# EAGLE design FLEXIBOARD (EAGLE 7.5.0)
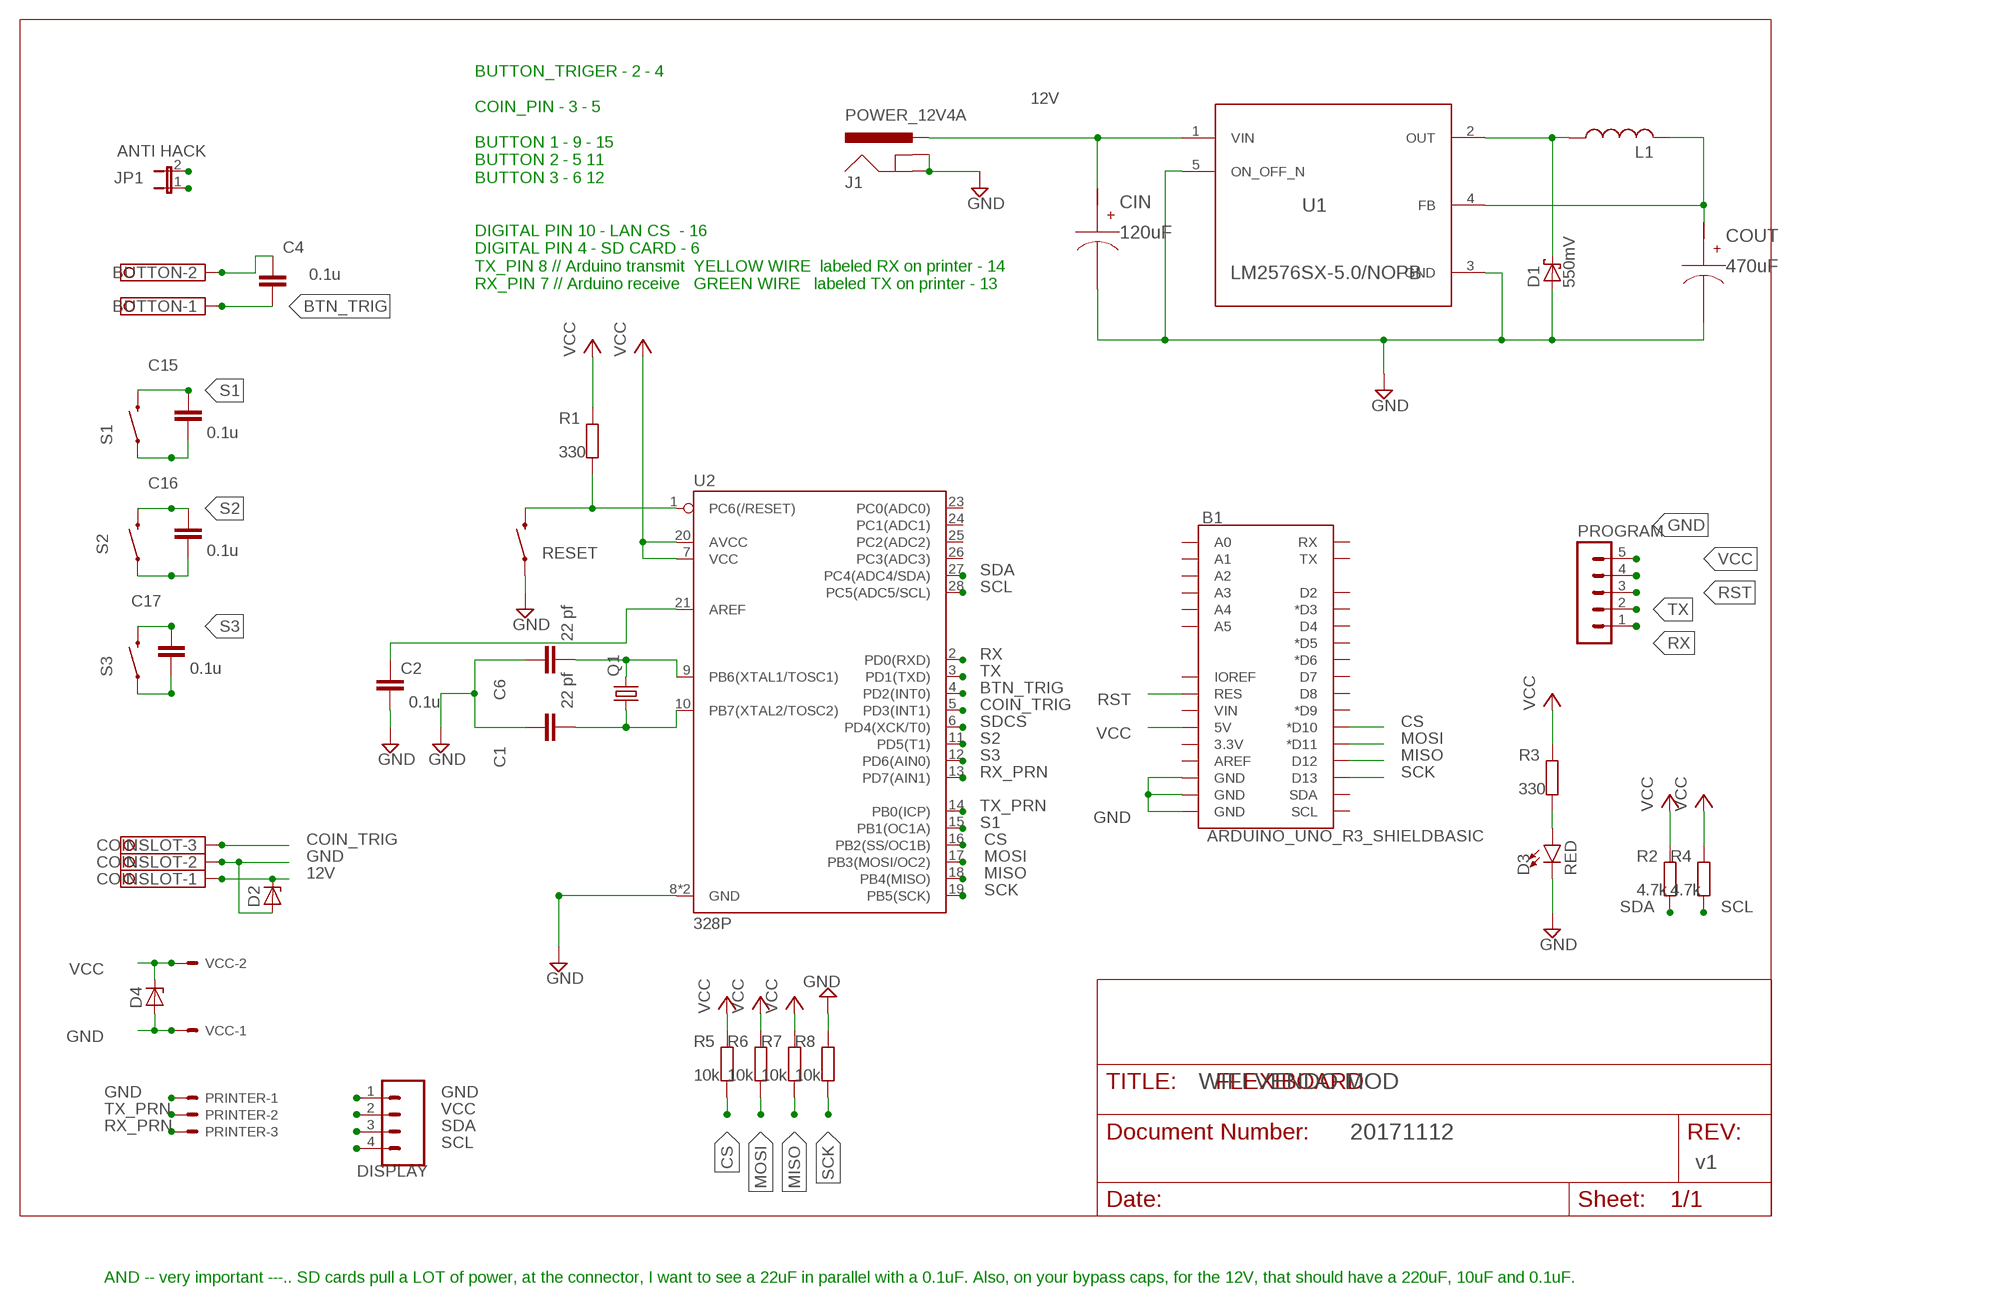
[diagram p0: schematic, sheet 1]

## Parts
B1  ARDUINO_UNO_R3_SHIELDBASIC  [UNO_R3_SHIELD]
BUTTON  TERMINAL-BLOCK-3.5MM-2-PIN-LONG-PAD  [TERMINAL-BLOCK-2-PIN-3.5MM-LONG-PAD]
C1  22 pf  C-EU050-024X044  [C050-024X044]
C2  0.1u  C-EU050-024X044  [C050-024X044]
C4  0.1u  C-EU050-024X044  [C050-024X044]
C6  22 pf  C-EU050-024X044  [C050-024X044]
C15  0.1u  C-EU050-024X044  [C050-024X044]
C16  0.1u  C-EU050-024X044  [C050-024X044]
C17  0.1u  C-EU050-024X044  [C050-024X044]
CIN  120uF  20SVPF120M  [CAPSMT_62_F61_T]
COINSLOT  TERMINAL-BLOCK-3.5MM-3-PIN-LONG-PAD  [TERMINAL-BLOCK-3-PIN-3.5MM-LONG-PAD]
COUT  470uF  EEE-FC1A471P  [SM_RADIAL_G_T]
D1  550mV  SCHOTTKY-DIODEC4111-15  [C4111-15]
D2  ZENER-DIODEF126-12  [F126Z12]
D3  RED  LED5MM  [LED_5MM]
D4  ZENER-DIODEF126-12  [F126Z12]
DISPLAY  M04PTH  [1X04]
J1  POWER_12V4A  POWER_JACKPTH  [POWER_JACK_PTH]
JP1  ANTI HACK  JUMPER-2SMD-NO  [SJ_2S-NO]
L1  L_USF  [INDUCTOR_CDRH127]
PRINTER  JST-XH-03-PIN-LONG-PAD  [JST-XH-03-PACKAGE-LONG-PAD]
PROGRAM  MA05-1  [MA05-1]
Q1  CRYSTALSM49  [SM49]
R1  330  R-EU_0204/7  [0204/7]
R2  4.7k  R-EU_0204/7  [0204/7]
R3  330  R-EU_0204/7  [0204/7]
R4  4.7k  R-EU_0204/7  [0204/7]
R5  10k  R-EU_0204/7  [0204/7]
R6  10k  R-EU_0204/7  [0204/7]
R7  10k  R-EU_0204/7  [0204/7]
R8  10k  R-EU_0204/7  [0204/7]
RESET  SWITCH-MOMENTARY-2PTH_EZ  [TACTILE-PTH-EZ]
S1  SWITCH-MOMENTARY-2PTH_EZ  [TACTILE-PTH-EZ]
S2  SWITCH-MOMENTARY-2PTH_EZ  [TACTILE-PTH-EZ]
S3  SWITCH-MOMENTARY-2PTH_EZ  [TACTILE-PTH-EZ]
U1  LM2576SX-5.0/NOPB  [KTT0005B_T]
U2  328P  ATMEGA328P_PDIP  [DIP28]
VCC  JST-XH-02-PIN-LONG-PAD  [JST-XH-02-PACKAGE-LONG-PAD]

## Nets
12V: CIN.P$1(+) COINSLOT.1 D2.C J1.PWR U1.1(VIN)
BTN_TRIG: BUTTON.1 C4.2 U2.4(PD2(INT0))
COIN_TRIG: COINSLOT.3 U2.5(PD3(INT1))
CS: B1.D10(*D10) R5.1 U2.16(PB2(SS/OC1B))
GND: B1.GND@0(GND) B1.GND@1(GND) B1.GND@2(GND) BUTTON.2 C1.1 C2.2 C4.1 C6.1 C15.2 C16.2 C17.2 CIN.P$2(-) COINSLOT.2 COUT.P$2(-) D1.A D2.A D3.K(C) D4.A DISPLAY.1 J1.GND J1.GNDBREAK PRINTER.1 PROGRAM.5 R8.2 RESET.1 S1.1 S2.1 S3.1 U1.3(GND) U1.5(ON_OFF_N) U2.8(GND) U2.22(GND) VCC.1
MISO: B1.D12 R7.1 U2.18(PB4(MISO))
MOSI: B1.D11(*D11) R6.1 U2.17(PB3(MOSI/OC2))
N$1: C6.2 Q1.2 U2.9(PB6(XTAL1/TOSC1))
N$2: C1.2 Q1.1 U2.10(PB7(XTAL2/TOSC2))
N$4: D1.C L1.1 U1.2(OUT)
N$6: D3.A R3.1
N$7: C2.1 U2.21(AREF)
RST: B1.RES PROGRAM.3 R1.1 RESET.3 U2.1(PC6(/RESET))
RX: JP1.2 PROGRAM.1 U2.2(PD0(RXD))
RX_PRN: PRINTER.3 U2.13(PD7(AIN1))
S1: C15.1 S1.3 U2.15(PB1(OC1A))
S2: C16.1 S2.3 U2.11(PD5(T1))
S3: C17.1 S3.3 U2.12(PD6(AIN0))
SCK: B1.D13 R8.1 U2.19(PB5(SCK))
SCL: DISPLAY.4 R4.1 U2.28(PC5(ADC5/SCL))
SDA: DISPLAY.3 R2.1 U2.27(PC4(ADC4/SDA))
SDCS: U2.6(PD4(XCK/T0))
TX: JP1.1 PROGRAM.2 U2.3(PD1(TXD))
TX_PRN: PRINTER.2 U2.14(PB0(ICP))
VCC: B1.5V COUT.P$1(+) D4.C DISPLAY.2 L1.2 PROGRAM.4 R1.2 R2.2 R3.2 R4.2 R5.2 R6.2 R7.2 U1.4(FB) U2.7(VCC) U2.20(AVCC) VCC.2
Unconnected: B1.3.3V B1.A0 B1.A1 B1.A2 B1.A3 B1.A4 B1.A5 B1.AREF B1.D2 B1.D3(*D3) B1.D4 B1.D5(*D5) B1.D6(*D6) B1.D7 B1.D8 B1.D9(*D9) B1.IOREF B1.RX B1.SCL B1.SDA B1.TX B1.VIN U2.23(PC0(ADC0)) U2.24(PC1(ADC1)) U2.25(PC2(ADC2)) U2.26(PC3(ADC3))

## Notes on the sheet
- BUTTON_TRIGER - 2 - 4
  
  COIN_PIN - 3 - 5
  
  BUTTON 1 - 9 - 15
  BUTTON 2 - 5 11
  BUTTON 3 - 6 12
  
  
  DIGITAL PIN 10 - LAN CS  - 16
  DIGITAL PIN 4 - SD CARD - 6
  TX_PIN 8 // Arduino transmit  YELLOW WIRE  labeled RX on printer - 14
  RX_PIN 7 // Arduino receive   GREEN WIRE   labeled TX on printer - 13
- WIFI VENDO MOD
- 20171112
- SCL
- v1
- AND -- very important ---.. SD cards pull a LOT of power, at the connector, I want to see a 22uF in parallel with a 0.1uF. Also, on your bypass caps, for the 12V, that should have a 220uF, 10uF and 0.1uF.

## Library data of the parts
B1 = SparkFun-Boards:ARDUINO_UNO_R3_SHIELD: Arduino R3 Shield Footprint Shield form compatible with the Arduino Uno R3. SparkFun Products: MG2639 Cellular Shield MIDI Shield R3 Stackable Headers Kit
BUTTON = Rembrandt Electronics - Terminal Block 3-5mm v1-0:TERMINAL-BLOCK-3.5MM-2-PIN: Terminal Block 3.5mm
C1 C2 C4 C6 C15-C17 = resistor:C-EU: CAPACITOR, European symbol
CIN = AcceleratedDesigns_Lib:20SVPF120M
COINSLOT = Rembrandt Electronics - Terminal Block 3-5mm v1-0:TERMINAL-BLOCK-3.5MM-3-PIN: Terminal Block 3.5mm Pitch: 3,5 mm Number of pins: 3 Created by Rembrandt Electronics www.rembrandtelectronics.com
COUT = AcceleratedDesigns_Lib:EEE-FC1A471P
D1 = diode:SCHOTTKY-DIODE: Schottky Diode
D2 D4 = diode:ZENER-DIODE: Z-Diode
D3 = SparkFun-LED:LED: LED (Generic)
DISPLAY = SparkFun-Connectors:M04: Header 4 Standard 4-pin 0.1" header. Use with straight break away headers (SKU : PRT-00116), right angle break away headers (PRT-00553), swiss pins (PRT-00743), machine pins (PRT-00117), and female headers (PRT-00115). Molex polarized connector foot print use with SKU : PRT-08231 with associated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; PROD_ID: CONN-09696
J1 = SparkFun-Connectors:POWER_JACK: Power Jack This is the standard 5.5mm barrel jack for power. The PTH is the most common, proven, reliable, footprint. The Slot footprint only works if the mill layer is transmitted to the PCB fab house so be warned. Mating wall wart : TOL-00298 (and others); PROD_ID: CONN-08197
JP1 = SparkFun-Retired:JUMPER-2: Jumper
L1 = m-pad-2.1:L_US: Inductors in various packages from:
PRINTER = Rembrandt Electronics - JST XH Connectors v1-0:JST-XH-03-PIN: JST XH Connector 2 Pin Wire to board connector. Pitch: 2,54 mm, (0.100") Number of pins: 3 Created by Rembrandt Electronics www.rembrandtelectronics.com
PROGRAM = con-lstb:MA05-1: PIN HEADER; OC_FARNELL: unknown; OC_NEWARK: unknown
Q1 = crystal:CRYSTAL: CRYSTAL; OC_FARNELL: unknown; OC_NEWARK: unknown
R1-R8 = resistor:R-EU_: RESISTOR, European symbol
RESET S1-S3 = SparkFun-Electromechanical:SWITCH-MOMENTARY-2: Various NO switches- pushbuttons, reed, etc
U1 = AcceleratedDesigns_Lib:LM2576SX-5.0/NOPB
U2 = SparkFun-IC-Microcontroller:ATMEGA328P_PDIP: Atmel 328P Through hole ATMEGA328P uC used in the Arduino 32kb flash, 1k EEPROM, 2k SRAM Datasheet SparkFun Products Storefront component: AVR 28 Pin 20MHz 32K 6A/D - ATMega328P (COM-09061) SparkFun Simon Says - Through-Hole Soldering Kit (KIT-10547) SparkFun Learn to Solder - Simon Says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; PROD_ID: IC-09136
VCC = Rembrandt Electronics - JST XH Connectors v1-0:JST-XH-02-PIN: JST XH Connector 2 Pin

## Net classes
0 default: width 0.406 mm

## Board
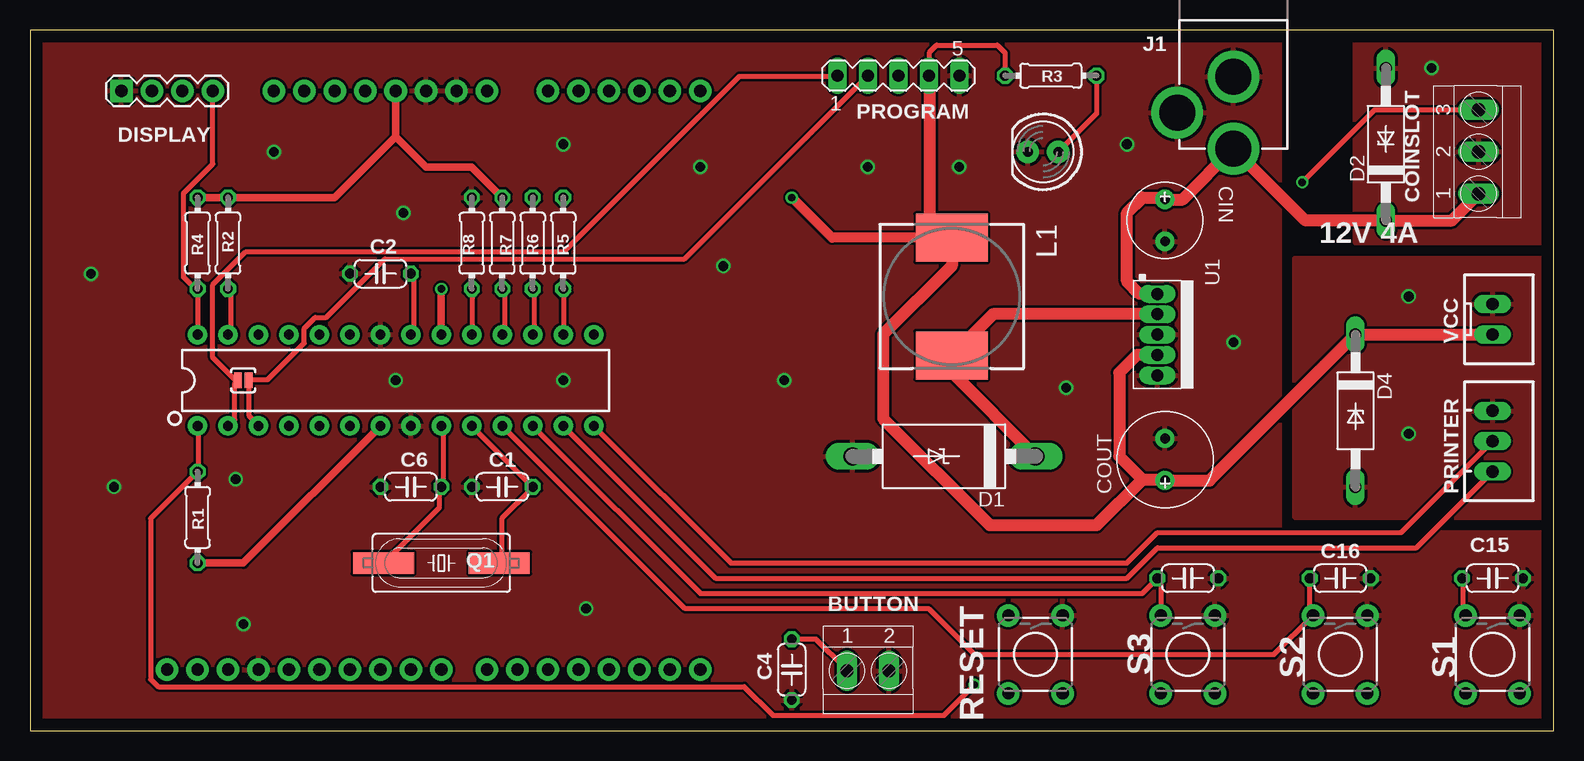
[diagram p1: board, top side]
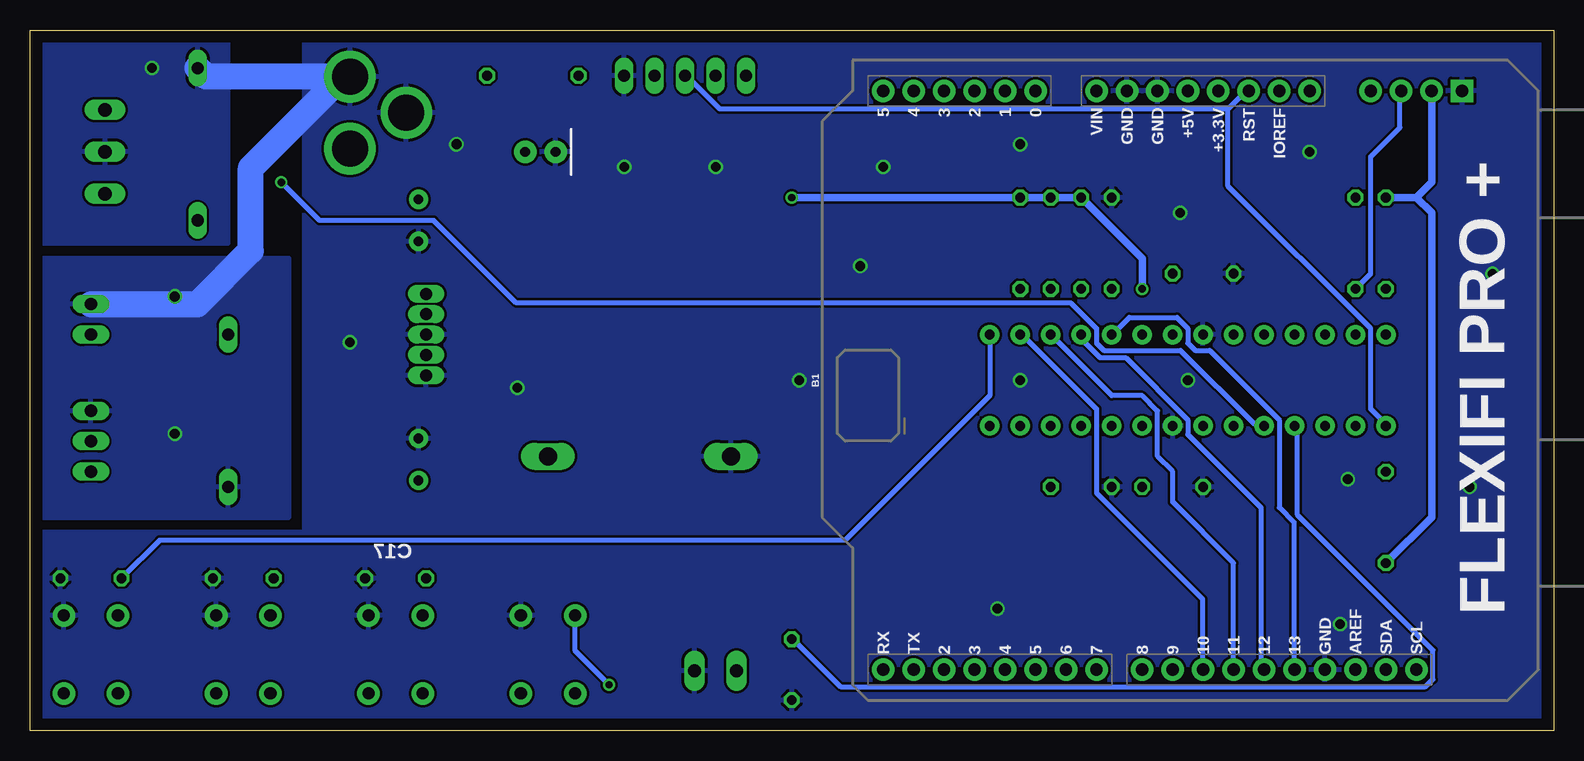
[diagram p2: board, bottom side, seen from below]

Size 127 x 58.42 mm. Coordinates in mm from the lower left corner, seen from the top.
Outline: 0,0 127,0 127,58.42 0,58.42 0,0
Copper layers (1*16): Top 0.035mm / dielectric 1.5mm / Bottom 0.035mm
Design rules "default *": minimum track width 10mil, minimum drill 24mil, track to track 8mil, track to pad 8mil, pad to pad 8mil, via to via 8mil, smd to smd 8mil, copper to edge 40mil, drill to drill 8mil, minimum pad ring 10mil, minimum via ring 8mil, stop-mask expansion 4mil, vias tented up to drill 0mil, thermal gap 10mil

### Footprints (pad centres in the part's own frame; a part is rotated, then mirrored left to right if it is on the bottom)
UNO_R3_SHIELD = drill 1.016 pad 1.88: 3.3V 24.13,-2.54; 5V 24.13,0; A0 24.13,12.7; A1 24.13,15.24; A2 24.13,17.78; A3 24.13,20.32; A4 24.13,22.86; A5 24.13,25.4; AREF -24.13,-13.97; D2 -24.13,20.32; D3 -24.13,17.78; D4 -24.13,15.24; D5 -24.13,12.7; D6 -24.13,10.16; D7 -24.13,7.62; D8 -24.13,3.81; D9 -24.13,1.27; D10 -24.13,-1.27; D11 -24.13,-3.81; D12 -24.13,-6.35; D13 -24.13,-8.89; GND@0 24.13,2.54; GND@1 24.13,5.08; GND@2 -24.13,-11.43; IOREF 24.13,-7.62; NC 24.13,-10.16; RES 24.13,-5.08; RX -24.13,25.4; SCL -24.13,-19.05; SDA -24.13,-16.51; TX -24.13,22.86; VIN 24.13,7.62
TERMINAL-BLOCK-2-PIN-3.5MM-LONG-PAD = drill 1.1 pad 1.7 long: 1 -1.75,-0.1; 2 1.75,-0.1
C050-024X044 = drill 0.813 octagon: 1 -2.54,0; 2 2.54,0
CAPSMT_62_F61_T = drill 0.8 pad 1.6: P$1 -1.75,0; P$2 1.75,0
TERMINAL-BLOCK-3-PIN-3.5MM-LONG-PAD = drill 1.1 pad 1.7 long: 1 -3.5,-0.1; 2 0,-0.1; 3 3.5,-0.1
SM_RADIAL_G_T = drill 0.8 pad 1.6: P$1 -1.75,0; P$2 1.75,0
C4111-15 = drill 1.499 long: A 7.62,0; C -7.62,0
F126Z12 = drill 1.016 long: A 6.35,0; C -6.35,0
LED_5MM = drill 0.813 pad 1.88: A -1.27,0; K 1.27,0
1X04 = drill 1.016 pad 1.88 square: 1 0,0 | drill 1.016 pad 1.88: 2 2.54,0; 3 5.08,0; 4 7.62,0
POWER_JACK_PTH = drill 2.997 pad 4.318: GND 0,7.7; GNDBREAK 4.7,10.7; PWR 0,13.7
SJ_2S-NO = smd 0.635 x 1.27: 1 -0.45,0; 2 0.45,0
INDUCTOR_CDRH127 = smd 6 x 4: 1 0,4.9; 2 0,-4.9
JST-XH-03-PACKAGE-LONG-PAD = drill 1.016 long: 1 -2.54,0; 2 0,0; 3 2.54,0
MA05-1 = drill 1.016 long: 1 -5.08,0; 2 -2.54,0; 3 0,0; 4 2.54,0; 5 5.08,0
SM49 = smd 5.08 x 1.778: 1 -4.826,0; 2 4.826,0
0204/7 = drill 0.813 octagon: 1 -3.81,0; 2 3.81,0
TACTILE-PTH-EZ = drill 1.016 pad 1.88: 1 -3.251,2.261; 2 3.251,2.261; 3 -3.251,-2.261; 4 3.251,-2.261
KTT0005B_T = drill 1 pad 1.27 long: 1 0,3.4; 2 0,1.7; 3 0,0; 4 0,-1.7; 5 0,-3.4
DIP28 = drill 0.813 pad 1.626: 1 -16.51,-3.81; 2 -13.97,-3.81; 3 -11.43,-3.81; 4 -8.89,-3.81; 5 -6.35,-3.81; 6 -3.81,-3.81; 7 -1.27,-3.81; 8 1.27,-3.81; 9 3.81,-3.81; 10 6.35,-3.81; 11 8.89,-3.81; 12 11.43,-3.81; 13 13.97,-3.81; 14 16.51,-3.81; 15 16.51,3.81; 16 13.97,3.81; 17 11.43,3.81; 18 8.89,3.81; 19 6.35,3.81; 20 3.81,3.81; 21 1.27,3.81; 22 -1.27,3.81; 23 -3.81,3.81; 24 -6.35,3.81; 25 -8.89,3.81; 26 -11.43,3.81; 27 -13.97,3.81; 28 -16.51,3.81
JST-XH-02-PACKAGE-LONG-PAD = drill 1.016 long: 1 -1.27,0; 2 1.27,0

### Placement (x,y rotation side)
B1  30.48,29.21 90 bottom
BUTTON  69.85,5.08 0 top
C1  39.37,20.32 0 top
C2  29.21,38.1 180 top
C4  63.5,5.08 90 top
C6  31.75,20.32 0 top
C15  121.92,12.7 0 top
C16  109.22,12.7 0 top
C17  96.52,12.7 0 top
CIN  94.61,42.55 270 top
COINSLOT  120.65,48.26 90 top
COUT  94.61,22.61 90 top
D1  76.2,22.86 180 top
D2  113.03,48.9 90 top
D3  84.45,48.26 180 top
D4  110.49,26.67 270 top
DISPLAY  7.62,53.34 0 top
J1  100.33,62.23 180 top
JP1  17.78,29.21 180 top
L1  76.83,36.2 180 top
PRINTER  121.92,24.13 270 top
PROGRAM  72.39,54.61 0 top
Q1  34.29,13.97 180 top
R1  13.97,17.78 270 top
R2  16.51,40.64 90 top
R3  85.09,54.61 180 top
R4  13.97,40.64 90 top
R5  44.45,40.64 90 top
R6  41.91,40.64 90 top
R7  39.37,40.64 90 top
R8  36.83,40.64 90 top
RESET  83.82,6.35 270 top
S1  121.92,6.35 270 top
S2  109.22,6.35 270 top
S3  96.52,6.35 270 top
U1  93.98,33.02 0 top
U2  30.48,29.21 0 top
VCC  121.92,34.29 270 top

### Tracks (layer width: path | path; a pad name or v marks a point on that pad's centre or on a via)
12V
  Top 1.016: COINSLOT.1 118.53,42.55 D2.C 106.31,42.55 J1.PWR 96.09,44.3 CIN.P$1 94.46,44.45 92.71,44.45 91.44,43.18 91.44,37.47 92.48,36.42 U1.1
BTN_TRIG
  Top 0.406: C4.2 65.53,7.62 67.97,5.18 BUTTON.1
  Bottom 0.406: U2.4 21.34,25.3 21.34,17.98 10.06,6.71 10.06,4.27 10.67,3.66 59.44,3.66 63.4,7.62 C4.2
COIN_TRIG  (via drill 0.6)
  Top 0.406: v106.05,45.72 112.08,51.76 COINSLOT.3
  Bottom 0.406: U2.5 24.38,25.6 24.99,25.6 31.09,31.7 37.49,31.7 38.1,32.31 38.1,33.53 40.23,35.66 86.46,35.66 93.34,42.55 102.87,42.55 v106.05,45.72
CS
  Top 0.406: R5.1 44.5,36.58 44.5,33.22 U2.16
  Bottom 0.406: B1.D10 29.26,5.18 29.26,10.97 38.1,19.81 38.1,26.82 44.2,32.92 U2.16
GND  (via drill 0.8)
  Bottom 2.184: J1.GND 100.97,54.53 | 100.97,54.53 112.31,54.53 D2.A | VCC.1 113.03,35.56 108.58,40.01 108.58,46.91 100.97,54.53
  other vias: 55.88,46.99 44.45,48.9 20.32,48.26 31.11,43.18 5.08,38.1 6.99,20.32 17.78,8.89 17.14,20.95 46.35,10.16 44.45,29.21 30.48,29.21 57.78,38.73 62.87,29.21 69.85,46.99 77.47,46.99 86.36,28.57 100.33,32.38 114.94,36.2 114.94,24.77 116.84,55.24 91.44,48.9
  pour Top: -31.75,69.85 104.14,69.85 104.14,16.51 138.43,16.51 138.43,-12.7 -31.75,-12.7
  pour Bottom: -25.4,63.5 104.14,63.5 104.14,16.51 132.08,16.51 132.08,-6.35 -25.4,-6.35
  pour Top: 130.81,39.37 105.41,39.37 105.41,17.78 130.81,17.78
  pour Bottom: 105.41,39.37 129.54,39.37 129.54,17.78 105.41,17.78
  pour Top: 110.49,40.64 110.49,59.69 130.81,59.69 130.81,40.64
  pour Bottom: 110.49,59.69 129.54,59.69 129.54,40.64 110.49,40.64
MISO
  Top 0.406: R7.1 39.62,36.58 39.62,33.22 U2.18
  Bottom 0.406: B1.D12 24.38,5.18 24.38,18.59 30.48,24.69 30.48,25.91 35.66,31.09 37.8,31.09 39.62,32.92 U2.18
MOSI
  Top 0.406: R6.1 42.06,36.58 42.06,33.22 U2.17
  Bottom 0.406: B1.D11 26.67,13.97 31.75,19.05 31.75,21.59 33.02,22.86 33.02,26.67 34.29,27.94 36.83,27.94 U2.17
N$1
  Top 0.406: U2.9 34.44,25.3 34.44,20.42 C6.2 34.14,20.12 34.14,18.59 29.57,14.02 Q1.2
N$2
  Top 0.406: U2.10 36.88,25.3 41.76,20.42 C1.2 41.76,20.12 39.32,17.68 39.32,14.02 Q1.1
N$4
  Top 1.016: D1.C 76.83,29.84 L1.1 80.26,34.72 U1.2
N$6
  Top 0.406: 89,54.56 R3.1 88.9,51.44 D3.A
N$7
  Top 0.406: C2.1 32,38.1 32,33.22 U2.21
RST  (via drill 0.6)
  Top 0.406: U2.1 14.02,25.3 14.02,21.64 R1.1 10.06,17.68 10.06,4.27 10.67,3.66 59.54,3.66 61.92,1.27 76.2,1.27 v78.74,3.81
  Bottom 0.406: 27.13,51.82 69.49,51.82 72.24,54.56 PROGRAM.3 | 27.13,51.82 25.6,53.34 B1.RES | 27.13,51.82 27.13,45.41 15.24,33.53 15.24,26.82 14.02,25.6 U2.1 | RESET.3 81.56,6.63 v78.74,3.81
RX
  Top 0.406: U2.2 16.76,25.6 17.07,25.91 17.07,28.96 JP1.2 17.07,29.26 15.24,31.09 15.24,37.19 17.98,39.93 44.5,39.93 59.13,54.56 67.06,54.56 PROGRAM.1
RX_PRN
  Top 0.406: U2.13 57.15,12.7 91.44,12.7 93.98,15.24 115.57,15.24 PRINTER.3
S1
  Top 0.406: C15.1 119.48,12.5 119.48,9.75 S1.3
  Bottom 0.406: U2.15 46.99,27.94 59.05,15.88 116.2,15.88 C15.1
S2
  Top 0.406: C16.1 106.68,9.75 S2.3 103.71,6.35 78.74,6.35 74.93,10.16 54.61,10.16 U2.11
S3
  Top 0.406: U2.12 55.88,11.43 92.71,11.43 C17.1 94.26,12.42 S3.3
SCK
  Top 0.406: R8.1 36.88,36.58 36.88,33.22 U2.19
  Bottom 0.406: B1.D13 21.64,5.18 21.64,17.37 22.86,18.59 22.86,25.91 28.65,31.7 29.87,31.7 30.48,32.31 30.48,33.53 31.39,34.44 35.36,34.44 36.58,33.22 U2.19
SCL
  Top 0.406: U2.28 14.02,33.22 14.02,36.58 R4.1 13.72,36.88 12.8,37.8 12.8,44.81 15.24,47.24 DISPLAY.4
SDA
  Top 0.406: R2.1 16.76,36.58 16.76,33.22 U2.27
  Bottom 0.406: R2.1 15.24,38.1 15.24,47.85 12.8,50.29 12.8,53.34 DISPLAY.3
TX
  Top 0.406: U2.3 18.9,25.6 18.29,26.21 18.29,28.96 JP1.1 18.29,29.26 19.81,29.26 22.86,32.31 22.86,33.53 23.77,34.44 24.69,34.44 29.57,39.32 54.56,39.32 PROGRAM.2
TX_PRN
  Top 0.406: U2.14 58.42,13.97 91.44,13.97 93.98,16.51 114.3,16.51 PRINTER.2
VCC  (via drill 0.6)
  Top 0.406: PROGRAM.4 74.98,54.56 74.98,56.57 75.56,57.15 80.64,57.15 81.28,56.52 R3.2
  Top 0.61: R7.2 36.83,46.99 33.02,46.99 30.48,49.53 | 30.48,49.53 B1.5V | R4.2 R2.2 25.4,44.45 30.48,49.53 | U2.7 17.78,13.97 R1.2 | U2.20 v34.29,36.83
  Top 0.813: L1.2 66.86,41.09 v63.5,44.45
  Top 1.016: 74.98,54.56 74.98,42.95 L1.2 76.83,38.73 71.12,33.02 71.12,26.04 80.01,17.14 88.9,17.14 92.71,20.95 | VCC.2 D4.C 98.33,20.86 COUT.P$1 94.52,20.95 92.71,20.95 | U1.4 92.28,31.32 90.81,29.84 90.81,22.86 92.71,20.95
  Bottom 0.406: 74.98,54.56 PROGRAM.4
  Bottom 0.61: v63.5,44.45 R5.2 R6.2 R7.2 34.29,39.37 v34.29,36.83 | R4.2 11.43,44.45 | 11.43,44.45 10.16,43.18 10.16,17.78 R1.2 | DISPLAY.2 10.16,45.72 11.43,44.45

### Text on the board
tPlace: 12V 4A
bPlace: FLEXIFI PRO +

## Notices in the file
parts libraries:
SparkFun-Electromechanical: Licensing: Creative Commons ShareAlike 4.0 International - https://creativecommons.org/licenses/by-sa/4.0
m-pad-2.1: License : GNU General Public License version 2 (see bottom)
